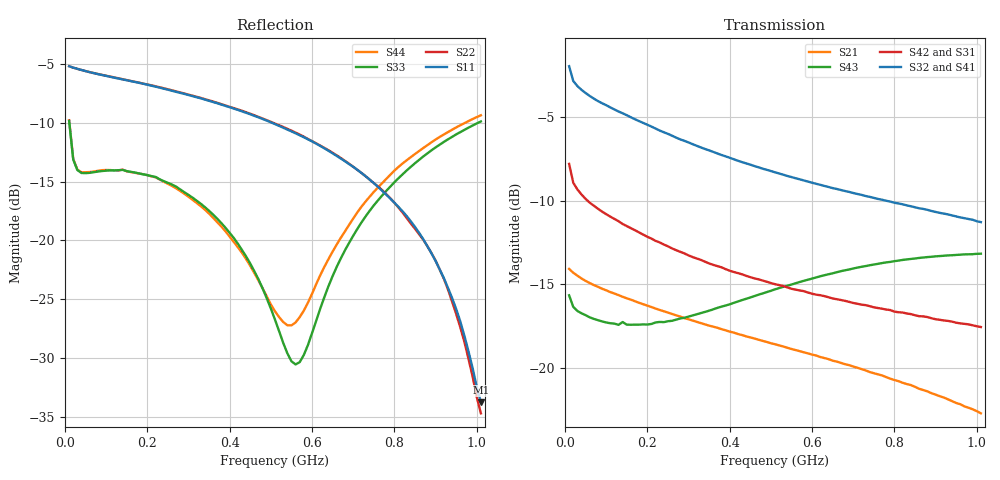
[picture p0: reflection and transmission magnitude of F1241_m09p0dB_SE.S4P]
! Integrated Device Technology
! Corporate Headquarters
! 6024 Silver Creek Valley Road
! San Jose, CA 95138  USA
! Phone:  1-408-284-8200
! Toll Free:  1-800-223-1366
! Webpage:  http://www.idt.com/
! Timing and RF Division
! 515 Groton Road, Suite 102
! Westford, MA 01886-6024
! Device:  F1241
! Description: Dual Intermediate Frequency Digital Variable Gain Amplifier
! Frequency:  10.0 -  500.00 MHz
! Package:  5x5 mm QFN Plastic Package: 32 pin
! Ports:  8 RF, 20 DC
!  Pin  1  = GA3  Pin 17  = RF OUT_B+
!  Pin  2  = GA4  Pin 18  = RF OUT_B-
!  Pin  3  = GA5  Pin 19  = STBY_B
!  Pin  4  = ISET_A  Pin 20  = Ground
!  Pin  5  = ISET_B  Pin 21  = Ground
!  Pin  6  = GB5  Pin 22  = STB_A
!  Pin  7  = GB4  Pin 23  = RF OUT_A-  = Port 4
!  Pin  8  = GB3  Pin 24  = RF OUT_A+  = Port 3
!  Pin  9  = GB2  Pin 25  = NO CONNECT
!  Pin 10  = GB1  Pin 26  = NO CONNECT
!  Pin 11  = RF IN_B+  Pin 27  = VCC
!  Pin 12  = RF IN_B-  Pin 28  = Ground
!  Pin 13  = Ground  Pin 29  = RF IN_A-  = Port 2
!  Pin 14  = VCC  Pin 30  = RF IN_A+  = Port 1
!  Pin 15  = NO CONNECT  Pin 31  = GA1
!  Pin 16  = NO CONNECT  Pin 32  = GA2
! State:  29
! Gain State:  -9.0 dB
! Voltages:  Vcc = +5.00 Volts  Icc approximately 160.0 mA or 80 mA per channel.
! Data:  The device was measured on a custom evaluation board which has
!  individual transmission lines to the RF pins.  Data was collected
!  using a calibrated network analyzer.  The evaluation board was
!  de-embedded using a port reference technique.
!  The reference plane is the edge of the package pin.
!  Only Channel A was measured.
!  This data is in single-ended operation.  If your needs are balanced
!  or differential S-parameters then this file needs to be used a
!  linear simulator.
! Misc:  Lot Code  160028MY
!  Action Tracker AT004
! Date Measured:  2014-08-14
! Date:  2014-08-28  MJV
! Note:
!  Integrated Device Technology supplies this data as a sample of measured
!  data at the package pin for this product.  Your particular data for this
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# Hz S dB R 50
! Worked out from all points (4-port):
!   101 points, 10 MHz to 1.01 GHz, reference 50 ohm
!   strongest paths, dB at 10 MHz, 260 MHz, 510 MHz, 760 MHz, 1.01 GHz:
!     S32: -1.9, -6.1, -8.3, -9.9, -11.3
!     S41: -1.9, -6.1, -8.4, -10.1, -11.6
!     S42: -7.8, -12.9, -15.0, -16.4, -17.6
!     S31: -7.8, -12.9, -15.1, -16.5, -17.6
!     S43: -15.7, -17.2, -15.3, -13.8, -13.2
!     S21: -14.1, -16.8, -18.6, -20.4, -22.7
!   lowest |S11| = -33.8 dB at 1.01 GHz (marker M1), VSWR 1.04, Z = 51.7 + j1.14 ohm
!   |S11| at or under -10 dB: 504.2 MHz to end of sweep
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1e7  -5.16 -4.1  -14.06 -8.3  -33.22 -2.5  -26.88 4.9
     -14.08 -8.2  -5.15 -4.0  -26.88 4.7  -33.20 -2.6
     -7.81 157.1  -1.95 165.1  -9.80 -45.1  -15.70 177.0
     -1.91 165.2  -7.80 157.3  -15.66 177.1  -9.76 -44.8
4e7  -5.48 -5.5  -14.63 -10.1  -33.97 -8.4  -27.26 -5.4
     -14.66 -10.1  -5.47 -5.3  -27.26 -5.1  -34.02 -8.5
     -9.64 156.6  -3.36 164.4  -14.25 -13.8  -16.80 167.2
     -3.32 164.2  -9.63 156.5  -16.74 167.2  -14.19 -13.4
3.8e8  -8.43 -17.1  -17.67 -34.5  -36.90 -10.0  -29.12 -18.6
       -17.69 -34.6  -8.39 -15.9  -28.95 -18.4  -36.86 -12.2
       -14.10 82.9  -7.26 120.5  -18.53 -9.6  -16.43 107.8
       -7.33 119.2  -13.99 82.0  -16.34 107.6  -18.82 -4.5
5.6e8  -10.87 -20.6  -18.91 -43.1  -36.65 -6.7  -29.17 -23.2
       -18.94 -43.2  -10.81 -19.2  -28.78 -23.7  -36.63 -9.2
       -15.43 54.5  -8.66 104.0  -30.56 56.1  -15.05 82.8
       -8.79 102.4  -15.33 53.0  -14.94 82.6  -26.98 68.2
7.1e8  -13.98 -22.7  -19.97 -49.9  -35.95 -6.1  -29.20 -28.4
       -20.00 -50.0  -13.98 -21.4  -28.56 -29.7  -35.97 -9.6
       -16.27 34.5  -9.60 91.2  -19.02 124.3  -14.14 63.6
       -9.80 89.7  -16.17 32.0  -14.01 63.4  -17.61 117.9
8.7e8  -19.89 -21.3  -21.26 -56.8  -35.05 -8.5  -29.23 -34.8
       -21.34 -56.9  -19.94 -21.5  -28.44 -36.8  -35.18 -11.2
       -17.03 16.0  -10.49 78.1  -12.85 124.8  -13.54 44.9
       -10.77 76.8  -16.93 12.7  -13.40 44.8  -12.13 120.9
1.01e9  -33.78 32.4  -22.65 -62.0  -34.31 -12.1  -29.34 -40.6
        -22.73 -62.2  -34.73 28.5  -28.34 -43.4  -34.29 -15.1
        -17.61 1.8  -11.28 66.9  -9.86 121.8  -13.32 30.4
        -11.58 66.1  -17.56 -2.2  -13.17 30.3  -9.33 118.1
